|   IBIS Model for OMAP-L138ZWT
[IBIS Ver]   3.2
[Comment Char]  |_char
[File Name]   omapl138_zwt.ibs
[File Rev]   1.0
[Date]   March 8, 2013
[Source]   From Optimal Corporation's PakSi-E result.
[Notes]   Created from Freon_16x16_OSV_12172008_H_1.mcm
|   (1) OMAP-L138 ZWT contains dual rail I/O buffers that
|   are capable of running are two different core
|   voltages depedent on the schematic hookup
|   (a) 1.8V
|   (b) 3.3V
|   (2) Specific Model Sections/Name Decoders are determined
|   based upon the value that is supplied to the
|   particular I/O buffer as well as any pull up/down
|   resistors that are selected. Refer to the Model Selecter
|   Definitions for details regarding model selection at
|   1.8V rail or the 3.3V rail.
[Disclaimer]
|   Please be aware that in the absence of a written agreement
|   Texas Instruments (TI) assumes no liability for:
|   (1) The accuracy of the IBIS models provided to your company
|   (2) The proper functioning of these Models in your design
|   or for any resulting applications;or
|   (3) Infringement of patents,copyrights, or intellectual
|   property rights resulting from your use of these models.
|   TI provides IBIS Models as a service to our customers and
|   therefore reserves the right to limit distribution of the
|   Models.
[Copyright] Copyright 2011, Texas Instruments Incorporated. All Rights Reserved
[Component]   OMAP-L138ZWT
[Manufacturer]   Texas Instruments
[Package]
| variable   typ   min   max
R_pkg   4.82714e-001  2.28452e-002  7.70788e-001
L_pkg   4.49415e-009  1.01960e-010  8.14120e-009
C_pkg   9.77617e-013  6.27144e-013  1.43784e-012
[Pin] signal_name  model_name R_pin   L_pin   C_pin
| Note: Signal Name(s) may be truncated to meet the 80 character
|  per line limit. Refer to the IBIS Specification v3.2 for details
|   Name   I/O Model Name   R_pin  L_pin  C_pin
A1   ACLKR_PRU0_R3020  BC1833DV40CTPBFZ   6.70522e-001 7.77430e-009 1.18111e-012
B1   ACLKX_PRU0_R3019  BC1833DV40CTPBFZ   5.95613e-001 7.11870e-009 1.10755e-012
C2   AFSR_GP013   BC1833DV40CTPBFZ   5.89537e-001 6.09860e-009 1.05275e-012
B2   AFSX_GP012   BC1833DV40CTPBFZ   6.03424e-001 6.46010e-009 1.17554e-012
A2   AHCLKR_PRU0   BC1833DV40CTPBFZ   7.35160e-001 8.00800e-009 1.28347e-012
A3   AHCLKX_USB_REFCL  BC1833DV40CTPBFZ   6.42625e-001 7.06830e-009 1.36079e-012
D5   AMUTE_PRU0_R3016  BC1833DV40CTPBFZ   4.86289e-001 4.23260e-009 1.27108e-012
F4   RTCALARM_UART2CTS BC1833DV40CTPBFZ   2.81206e-001 2.78020e-009 1.04628e-012
F3   AXR0_ECAP0_APWM0  BC1833DV40CTPBFZ   4.75476e-001 4.39770e-009 9.49020e-013
E1   AXR1_DX0_GP19   BC1833DV40CTPBFZ   5.93339e-001 6.18190e-009 8.74765e-013
D4   AXR10_DR1_GP02   BC1833DV40CTPBFZ   4.51090e-001 3.95820e-009 1.11813e-012
C5   AXR11_FSX1_GP03   BC1833DV40CTPBFZ   3.47764e-001 4.08280e-009 1.06988e-012
C4   AXR12_FSR1_GP04   BC1833DV40CTPBFZ   5.63347e-001 5.37170e-009 1.17818e-012
B3   AXR13_CLKX1_GP05  BC1833DV40CTPBFZ   5.67122e-001 5.57030e-009 1.00192e-012
B4   AXR14_CLKR1_GP06  BC1833DV40CTPBFZ   5.99370e-001 6.02370e-009 1.15465e-012
A4   AXR15_EPWM0TZ0   BC1833DV40CTPBFZ   6.42602e-001 6.52960e-009 1.05664e-012
E2   AXR2_DR0_GP110   BC1833DV40CTPBFZ   5.58852e-001 5.75040e-009 9.93021e-013
E3   AXR3_FSX0_GP111   BC1833DV40CTPBFZ   5.43755e-001 5.35620e-009 1.08545e-012
D1   AXR4_FSR0_GP112   BC1833DV40CTPBFZ   6.02267e-001 6.21600e-009 9.81175e-013
D3   AXR5_CLKX0_GP113  BC1833DV40CTPBFZ   5.70240e-001 5.75810e-009 1.11536e-012
C1   AXR6_CLKR0_GP114  BC1833DV40CTPBFZ   6.53337e-001 6.85970e-009 1.03127e-012
D2   AXR7_EPWM1TZ0   BC1833DV40CTPBFZ   5.67627e-001 5.78120e-009 1.00529e-012
E4   AXR8_CLKS1_ECAP1  BC1833DV40CTPBFZ   6.23878e-001 5.57980e-009 1.16291e-012
C3   AXR9_DX1_GP01   BC1833DV40CTPBFZ   5.40131e-001 5.24750e-009 1.09974e-012
C14  EMAA0_GP50   BC1833DV40CTPBFZ   4.25288e-001 4.03200e-009 8.58918e-013
D15  EMAA1_GP51   BC1833DV40CTPBFZ   6.48857e-001 6.26150e-009 1.03443e-012
C12  EMAA10_PRU1R3018  BC1833DV40CTPBFZ   4.43266e-001 3.29860e-009 9.62048e-013
B12  EMAA11_PRU1R3019  BC1833DV40CTPBFZ   4.58807e-001 4.50390e-009 8.92001e-013
D13  EMAA12_PRU1R3020  BC1833DV40CTPBFZ   5.70361e-001 5.18860e-009 1.11139e-012
D11  EMAA13_PRU0R3021  BC1833DV40CTPBFZ   2.99405e-001 2.17920e-009 8.54180e-013
A12  EMAA14_MMCSD0DAT7 BC1833DV40CTPBFZ   4.83438e-001 4.55840e-009 8.59351e-013
C11  EMAA15_MMCSD0DAT6 BC1833DV40CTPBFZ   4.98593e-001 4.57870e-009 9.76252e-013
E12  EMAA16_MMCSD0DAT5 BC1833DV40CTPBFZ   5.62236e-001 4.38610e-009 1.25589e-012
B11  EMAA17_MMCSD0DAT4 BC1833DV40CTPBFZ   5.53553e-001 5.27900e-009 9.29416e-013
E11  EMAA18_MMCSD0DAT3 BC1833DV40CTPBFZ   4.25775e-001 3.44230e-009 1.11095e-012
C10  EMAA19_MMCSD0DAT2 BC1833DV40CTPBFZ   3.59339e-001 3.13160e-009 8.65773e-013
B14  EMAA2_GP52   BC1833DV40CTPBFZ   4.90044e-001 4.46920e-009 8.58488e-013
A11  EMAA20_MMCSD0DAT1 BC1833DV40CTPBFZ   5.00066e-001 4.69570e-009 8.08773e-013
B10  EMAA21_MMCSD0DAT0 BC1833DV40CTPBFZ   4.03175e-001 3.79000e-009 8.37205e-013
A10  EMAA22_MMCSD0CMD  BC1833DV40CTPBFZ   4.79165e-001 4.38050e-009 7.51561e-013
E9   MMCSD0CLK_GP47   BC1833DV40CTPBFZ   3.19355e-001 2.48480e-009 1.02209e-012
D14  EMAA3_GP53   BC1833DV40CTPBFZ   4.12224e-001 3.83380e-009 9.03674e-013
A14  EMAA4_GP54   BC1833DV40CTPBFZ   5.22455e-001 4.90270e-009 8.26256e-013
C13  EMAA5_GP55   BC1833DV40CTPBFZ   4.50260e-001 3.65480e-009 9.09443e-013
E13  EMAA6_GP56   BC1833DV40CTPBFZ   3.88312e-001 3.04460e-009 9.87596e-013
B13  EMAA7_PRU1R3015   BC1833DV40CTPBFZ   4.50502e-001 3.95110e-009 8.24200e-013
A13  EMAA8_PRU1R3016   BC1833DV40CTPBFZ   4.86150e-001 4.52080e-009 8.53585e-013
D12  EMAA9_PRU1R3017   BC1833DV40CTPBFZ   3.45739e-001 2.59770e-009 9.45330e-013
C15  EMABA0_GP28   BC1833DV40CTPBFZ   5.40104e-001 5.41780e-009 1.01378e-012
A15  EMABA1_GP29   BC1833DV40CTPBFZ   5.46634e-001 5.32220e-009 8.41073e-013
A9   EMACAS_PRU0R302   BC1833DV40CTPBFZ   4.68477e-001 4.48480e-009 7.79223e-013
B7   EMACLK_PRU0R305   BC1833DV40CTPBFZ   2.91044e-001 3.06540e-009 7.71567e-013
A18  EMACS0_GP20   BC1833DV40CTPBFZ   5.38591e-001 5.53120e-009 9.41554e-013
B17  EMACS2_GP315   BC1833DV40CTPBFZ   4.97514e-001 4.71050e-009 1.06659e-012
A17  EMACS3_GP314   BC1833DV40CTPBFZ   5.17167e-001 5.33980e-009 9.74323e-013
F9   EMA_CS4_GP313   BC1833DV40CTPBFZ   4.25846e-001 3.22730e-009 1.05377e-012
B16  EMA_CS5_GP312   BC1833DV40CTPBFZ   5.13656e-001 5.27280e-009 9.94069e-013
C9   EMA_D0_GP48   BC1833DV40CTPBFZ   2.94182e-001 2.42780e-009 7.80729e-013
A8   EMA_D1_GP49   BC1833DV40CTPBFZ   4.53721e-001 3.97270e-009 6.68142e-013
A7   EMA_D10_GP32   BC1833DV40CTPBFZ   4.53897e-001 4.01310e-009 6.27144e-013
D6   EMA_D11_GP33   BC1833DV40CTPBFZ   2.38604e-001 1.84040e-009 9.19954e-013
A6   EMA_D12_GP34   BC1833DV40CTPBFZ   6.07425e-001 6.23350e-009 1.06419e-012
B6   EMA_D13_GP35   BC1833DV40CTPBFZ   5.18704e-001 3.99570e-009 1.13613e-012
C7   EMA_D14_GP36   BC1833DV40CTPBFZ   5.42315e-001 4.44590e-009 1.15928e-012
E6   EMA_D15_GP37   BC1833DV40CTPBFZ   2.06956e-001 1.69280e-009 1.11364e-012
B8   EMA_D2_GP410   BC1833DV40CTPBFZ   4.73441e-001 3.98830e-009 7.85717e-013
E8   EMA_D3_GP411   BC1833DV40CTPBFZ   4.22749e-001 3.94410e-009 1.12372e-012
B5   EMA_D4_GP412   BC1833DV40CTPBFZ   4.51845e-001 3.85460e-009 8.63651e-013
E7   EMA_D5_GP413   BC1833DV40CTPBFZ   3.33586e-001 2.90310e-009 1.43784e-012
C6   EMA_D6_GP414   BC1833DV40CTPBFZ   4.96088e-001 3.85350e-009 1.08802e-012
D7   EMA_D7_GP415   BC1833DV40CTPBFZ   5.38361e-001 4.46010e-009 1.14437e-012
E10  EMA_D8_GP30   BC1833DV40CTPBFZ   4.32262e-001 3.32570e-009 1.05394e-012
D9   EMA_D9_GP31   BC1833DV40CTPBFZ   3.85347e-001 2.99080e-009 8.85071e-013
B15  EMA_OE_GP310   BC1833DV40CTPBFZ   4.72394e-001 4.44610e-009 9.78222e-013
A16  EMARAS_PRU0R303   BC1833DV40CTPBFZ   5.02224e-001 5.36240e-009 9.17657e-013
D10  EMA_A_RW_GP39   BC1833DV40CTPBFZ   4.33366e-001 3.89220e-009 1.09829e-012
D8   EMASDCKE_PRU0R304 BC1833DV40CTPBFZ   3.50532e-001 3.43390e-009 9.99262e-013
B18  EMAWAIT0_PRU0R300 BC1833DV40CTPBFZ   5.00826e-001 5.00220e-009 1.02162e-012
B19  EMAWAIT1_PRU0R301 BC1833DV40CTPBFZ   5.87512e-001 6.06000e-009 1.14362e-012
B9   EMAWE_GP311   BC1833DV40CTPBFZ   4.59931e-001 4.00200e-009 8.81437e-013
C8   EMAWEN_DQM0_GP23  BC1833DV40CTPBFZ   4.26501e-001 3.88670e-009 8.47385e-013
A5   EMAWEN_DQM1_GP22  BC1833DV40CTPBFZ   5.02300e-001 4.62500e-009 9.18201e-013
U7   DDR_A0   BSSTL18TCSCGPBFZ   4.45631e-001 3.19210e-009 8.01643e-013
T7   DDR_A1   BSSTL18TCSCGPBFZ   4.96539e-001 3.76940e-009 8.49415e-013
W6   DDR_A2   BSSTL18TCSCGPBFZ   4.96471e-001 4.42250e-009 7.26808e-013
V6   DDR_A3   BSSTL18TCSCGPBFZ   3.12088e-001 3.23310e-009 8.95189e-013
U5   DDR_A4   BSSTL18TCSCGPBFZ   5.26530e-001 4.12820e-009 9.39252e-013
V5   DDR_A5   BSSTL18TCSCGPBFZ   5.14992e-001 4.12960e-009 9.22902e-013
W5   DDR_A6   BSSTL18TCSCGPBFZ   5.19100e-001 4.88150e-009 7.93247e-013
U6   DDR_A7   BSSTL18TCSCGPBFZ   2.51410e-001 2.52800e-009 7.93128e-013
U4   DDR_A8   BSSTL18TCSCGPBFZ   6.12082e-001 5.53420e-009 1.02068e-012
T6   DDR_A9   BSSTL18TCSCGPBFZ   2.31771e-001 2.10850e-009 9.12907e-013
W4   DDR_A10   BSSTL18TCSCGPBFZ   5.78537e-001 5.31210e-009 8.57850e-013
T4   DDR_A11   BSSTL18TCSCGPBFZ   6.10590e-001 5.44020e-009 1.07076e-012
V4   DDR_A12   BSSTL18TCSCGPBFZ   5.44157e-001 4.83840e-009 8.98639e-013
T5   DDR_A13   BSSTL18TCSCGPBFZ   2.67446e-001 2.33590e-009 9.47633e-013
V8   DDR_BA0   BSSTL18TCSCGPBFZ   4.42216e-001 3.50310e-009 7.33337e-013
T9   DDR_BA1   BSSTL18TCSCGPBFZ   2.04349e-001 1.84940e-009 9.12926e-013
U8   DDR_BA2   BSSTL18TCSCGPBFZ   4.37893e-001 3.05980e-009 7.91011e-013
U9   DDR_CAS   BSSTL18TCSCGPBFZ   4.32382e-001 3.03600e-009 7.82466e-013
V7   DDR_CKE   BSSTL18TCSCGPBFZ   3.40193e-001 3.02880e-009 9.57595e-013
W7   DDR_CLKN   BSSTL18TCSCGPBFZ   4.87824e-001 4.14380e-009 7.11675e-013
W8   DDR_CLKP   BSSTL18TCSCGPBFZ   4.87706e-001 4.04160e-009 6.90005e-013
V9   DDR_CS   BSSTL18TCSCGPBFZ   4.22988e-001 3.32520e-009 7.05256e-013
U15  DDR_D0   BSSTL18TCSCGPBFZ   6.14599e-001 5.57430e-009 1.29241e-012
U14  DDR_D1   BSSTL18TCSCGPBFZ   6.77148e-001 6.88480e-009 1.15168e-012
V14  DDR_D2   BSSTL18TCSCGPBFZ   5.94668e-001 5.57310e-009 9.65300e-013
U13  DDR_D3   BSSTL18TCSCGPBFZ   6.42634e-001 6.44770e-009 1.01003e-012
V13  DDR_D4   BSSTL18TCSCGPBFZ   4.33037e-001 3.98350e-009 9.49332e-013
V12  DDR_D5   BSSTL18TCSCGPBFZ   5.17811e-001 4.36040e-009 8.60120e-013
W12  DDR_D6   BSSTL18TCSCGPBFZ   5.06957e-001 4.65170e-009 7.75559e-013
W11  DDR_D7   BSSTL18TCSCGPBFZ   3.40053e-001 3.84150e-009 8.42329e-013
T13  DDR_D8   BSSTL18TCSCGPBFZ   7.02824e-001 6.76610e-009 1.10155e-012
T11  DDR_D9   BSSTL18TCSCGPBFZ   5.38116e-001 4.19250e-009 9.33339e-013
T10  DDR_D10   BSSTL18TCSCGPBFZ   2.04836e-001 1.48950e-009 9.32683e-013
T12  DDR_D11   BSSTL18TCSCGPBFZ   5.39560e-001 4.18730e-009 9.72172e-013
U10  DDR_D12   BSSTL18TCSCGPBFZ   4.90524e-001 3.70090e-009 8.22331e-013
V10  DDR_D13   BSSTL18TCSCGPBFZ   5.08659e-001 4.15820e-009 8.09492e-013
U11  DDR_D14   BSSTL18TCSCGPBFZ   6.41945e-001 6.15820e-009 1.03041e-012
W10  DDR_D15   BSSTL18TCSCGPBFZ   3.34786e-001 3.81520e-009 1.10872e-012
W13  DDR_DQM0   BSSTL18TCSCGPBFZ   5.20588e-001 4.86740e-009 8.32828e-013
R10  DDR_DQM1   BSSTL18TCSCGPBFZ   5.83727e-001 4.04600e-009 1.10450e-012
W9   DDR_RAS   BSSTL18TCSCGPBFZ   4.85812e-001 4.18190e-009 7.68725e-013
R11  DDR_DQGATE0   BSSTL18TCSCGPBFZ   5.83676e-001 4.67250e-009 1.10827e-012
R12  DDR_DQGATE1   BSSTL18TCSCGPBFZ   6.09492e-001 4.92430e-009 1.16221e-012
T8   DDR_WE   BSSTL18TCSCGPBFZ   4.85661e-001 3.30550e-009 8.77513e-013
T14  DDR_DQS0   BSSTL18TCSCGPBFZ   5.56352e-001 4.85410e-009 1.06523e-012
V11  DDR_DQS1   BSSTL18TCSCGPBFZ   5.57030e-001 5.17590e-009 8.65934e-013
J16  EMU0   BC1833DV40CTPBFZ   2.69609e-001 2.51080e-009 9.18189e-013
K16  EMU1   BC1833DV40CTPBFZ   4.38711e-001 3.98660e-009 9.93256e-013
K4   PRU1R300_GP61   BC1833DV40CTPBFZ   3.74055e-001 3.00300e-009 9.72837e-013
J3   MMCSD1DAT1_GP62   BC1833DV40CTPBFZ   3.47731e-001 3.56010e-009 1.13728e-012
K3   MMCSD1DAT2_GP63   BC1833DV40CTPBFZ   4.24020e-001 3.61250e-009 8.08369e-013
H3   MMCSD1DAT3_GP64   BC1833DV40CTPBFZ   4.58330e-001 4.27570e-009 1.14982e-012
F2   MMCSD1DAT6_GP810  BC1833DV40CTPBFZ   6.57130e-001 6.53900e-009 1.00913e-012
F1   MMCSD1DAT7_GP811  BC1833DV40CTPBFZ   5.88435e-001 6.09970e-009 9.74970e-013
G3   PRU0R3022_GP812   BC1833DV40CTPBFZ   5.69940e-001 5.39570e-009 1.05523e-012
J4   PRU0R3023_GP813   BC1833DV40CTPBFZ   4.77184e-001 3.73550e-009 9.74249e-013
G2   PRU0R3024_GP814   BC1833DV40CTPBFZ   6.21314e-001 5.98450e-009 1.11595e-012
G1   PRU0R3025_GP815   BC1833DV40CTPBFZ   5.69099e-001 5.59150e-009 9.76024e-013
G4   MMCSD1DAT4_GP88   BC1833DV40CTPBFZ   4.94773e-001 4.21470e-009 9.49852e-013
H4   MMCSD1DAT5_GP89   BC1833DV40CTPBFZ   4.03091e-001 3.39770e-009 8.67477e-013
R5   GP60_PRU1_R3128   BC1833DV40CTPBFZ   2.17019e-001 2.01170e-009 1.03367e-012
W1   GP78_PRU1_R318   BC1833DV40CTPBFZ   6.10612e-001 6.27700e-009 1.06224e-012
W2   GP79_PRU1_R319   BC1833DV40CTPBFZ   6.30960e-001 6.09510e-009 1.07989e-012
T2   GP72_BOOT2   BC1833DV40CTPBFZ   5.01419e-001 4.54420e-009 9.41778e-013
T3   GP73_BOOT3   BC1833DV40CTPBFZ   4.48620e-001 3.96710e-009 1.00841e-012
R1   GP74_BOOT4   BC1833DV40CTPBFZ   5.49394e-001 5.30490e-009 8.92921e-013
R2   GP75_BOOT5   BC1833DV40CTPBFZ   5.25084e-001 4.72090e-009 9.30217e-013
R3   GP76_BOOT6   BC1833DV40CTPBFZ   3.55031e-001 4.19040e-009 1.05191e-012
P4   GP77_BOOT7   BC1833DV40CTPBFZ   4.27865e-001 3.34850e-009 9.06244e-013
W3   GP710_PRU1_R3110  BC1833DV40CTPBFZ   2.28452e-002 1.01960e-010 1.14444e-012
V1   GP711_PRU1_R3111  BC1833DV40CTPBFZ   6.46932e-001 6.50160e-009 9.88236e-013
V2   GP712_PRU1_R3112  BC1833DV40CTPBFZ   6.09370e-001 5.95910e-009 1.01546e-012
V3   GP713_PRU1_R3113  BC1833DV40CTPBFZ   5.28937e-001 5.19450e-009 1.02431e-012
U1   GP714_PRU1_R3114  BC1833DV40CTPBFZ   6.13427e-001 6.07030e-009 9.50946e-013
U2   GP715_PRU1_R3115  BC1833DV40CTPBFZ   5.67068e-001 5.44350e-009 9.82215e-013
U3   GP70_BOOT0   BC1833DV40CTPBFZ   5.43323e-001 4.88320e-009 9.28297e-013
T1   GP71_BOOT1   BC1833DV40CTPBFZ   5.55285e-001 5.17990e-009 8.95632e-013
J17  NMI   IC1833DVTPBFZP18LL 3.90575e-001 3.53870e-009 8.65772e-013
K14  RESET   IHHV1833DVTP18   2.72523e-001 1.96490e-009 1.01740e-012
K17  RTCK_GPIO80   BC1833DV40CTPBFZ   4.92642e-001 4.55900e-009 9.97242e-013
D19  SPI0CLK_EPWM0A   BC1833DV40CTPBFZ   4.59265e-001 4.70770e-009 8.79586e-013
C17  SPI0ENA_EPWM0B   BC1833DV40CTPBFZ   3.70510e-001 3.41200e-009 9.82922e-013
D17  SPI0SCS0_GP16   BC1833DV40CTPBFZ   4.89709e-001 4.51290e-009 9.79226e-013
E16  SPI0SCS1_GP17   BC1833DV40CTPBFZ   2.89181e-001 2.59760e-009 9.34814e-013
D16  SPI0SCS2_UART0RTS BC1833DV40CTPBFZ   3.74659e-001 3.47800e-009 1.02901e-012
E17  SPI0SCS3_UART0CTS BC1833DV40CTPBFZ   4.07379e-001 3.42510e-009 8.91820e-013
D18  SPI0SCS4_UART0TXD BC1833DV40CTPBFZ   4.05970e-001 4.12160e-009 9.47389e-013
C19  SPI0SCS5_UART0RXD BC1833DV40CTPBFZ   5.18855e-001 5.40240e-009 1.03877e-012
C18  SPI0SIMO_EPWMSYNO BC1833DV40CTPBFZ   4.65679e-001 4.70460e-009 9.61861e-013
C16  SPI0SOMI_EPWMSYNI BC1833DV40CTPBFZ   3.23590e-001 2.82350e-009 1.01704e-012
G19  SPI1CLK_GP213   BC1833DV40CTPBFZ   4.82388e-001 4.87790e-009 7.93438e-013
H16  SPI1ENA_GP212   BC1833DV40CTPBFZ   2.72059e-001 2.46120e-009 8.55327e-013
E19  SPI1SCS0_EPWM1B   BC1833DV40CTPBFZ   5.54124e-001 5.35800e-009 9.27298e-013
F18  SPI1SCS1_EPWM1A   BC1833DV40CTPBFZ   4.85756e-001 4.43690e-009 8.32222e-013
F19  SPI1SCS2_UART1TXD BC1833DV40CTPBFZ   5.30911e-001 5.08600e-009 7.97381e-013
E18  SPI1SCS3_UART1RXD BC1833DV40CTPBFZ   4.68304e-001 4.29180e-009 9.40515e-013
F16  SPI1SCS4_UART2TXD BC1833DV40CTPBFZ   3.84822e-001 3.09280e-009 8.50042e-013
F17  SPI1SCS5_UART2RXD BC1833DV40CTPBFZ   3.97204e-001 3.45760e-009 8.68842e-013
G18  SPI1SCS6_I2C0SDA  BC1833DV40CTPBFZ   4.36493e-001 3.97070e-009 8.05354e-013
G16  SPI1SCS7_I2C0SCL  BC1833DV40CTPBFZ   3.28582e-001 2.93800e-009 8.59756e-013
G17  SPI1SIMO_GP210   BC1833DV40CTPBFZ   4.15146e-001 3.62330e-009 7.78290e-013
H17  SPI1SOMI_GP211   BC1833DV40CTPBFZ   3.86238e-001 3.40470e-009 7.95949e-013
J15  TCK   IC1833DVTPBFZP18LL 2.72627e-001 2.07350e-009 9.10142e-013
M16  TDI   IC1833DVTPBFZP18LL 4.76009e-001 4.06980e-009 1.10114e-012
J18  TDO   BC1833DV40CTPBFZ   4.62219e-001 4.41060e-009 8.33533e-013
L16  TMS   IC1833DVTPBFZP18LL 4.14469e-001 3.71980e-009 9.85935e-013
L17  TRST   IC1833DVTPBFZP18LL 4.62541e-001 4.28940e-009 9.92132e-013
T17  RESETOUT_GP615   BC1833DV40CTPBFZ   3.51998e-001 3.17240e-009 1.08276e-012
U17  PRU0_R3029_GP611  BC1833DV40CTPBFZ   7.12182e-001 6.64690e-009 1.37972e-012
W15  PRU0_R3028_GP610  BC1833DV40CTPBFZ   5.66822e-001 5.43060e-009 8.83116e-013
W14  PRU1_R3010_GP67   BC1833DV40CTPBFZ   4.65680e-001 4.58120e-009 9.12942e-013
P17  GP65_PRU1_R310   BC1833DV40CTPBFZ   3.94808e-001 3.89780e-009 1.00392e-012
R15  PRU0R309_PRU0R319 BC1833DV40CTPBFZ   2.93369e-001 2.38090e-009 8.58888e-013
W17  RMIIRXER   BC1833DV40CTPBFZ   6.23033e-001 6.29800e-009 1.04906e-012
V17  RMIIRXD0   BC1833DV40CTPBFZ   6.63187e-001 6.71370e-009 1.15741e-012
W16  RMIIRXD1   BC1833DV40CTPBFZ   5.88099e-001 5.77390e-009 1.00930e-012
R14  RMIITXEN   BC1833DV40CTPBFZ   2.79926e-001 2.37250e-009 1.10763e-012
V16  RMIITXD0   BC1833DV40CTPBFZ   6.28546e-001 6.07180e-009 1.03347e-012
U18  RMIITXD1   BC1833DV40CTPBFZ   7.70788e-001 8.14120e-009 1.27165e-012
R19  PRU0R3010   BC1833DV40CTPBFZ   5.06077e-001 5.39890e-009 9.20909e-013
R18  PRU0R3011   BC1833DV40CTPBFZ   4.14016e-001 4.19930e-009 9.20996e-013
T16  PRU0R3012   BC1833DV40CTPBFZ   4.21661e-001 4.35600e-009 1.28119e-012
U19  PRU0R3013   BC1833DV40CTPBFZ   7.62887e-001 7.98930e-009 1.25280e-012
V19  PRU0R3014   BC1833DV40CTPBFZ   7.40621e-001 7.53910e-009 1.22918e-012
V18  PRU0R3015   BC1833DV40CTPBFZ   6.75889e-001 6.81150e-009 1.16111e-012
W19  RMIICRSDV   BC1833DV40CTPBFZ   7.15571e-001 7.47710e-009 1.14295e-012
W18  RMIIMHZ50CLK   BC1833DV40CTPBFZ   6.75324e-001 6.97490e-009 1.15470e-012
V15  PRU1R309_GP66   BC1833DV40CTPBFZ   3.14880e-001 3.37620e-009 8.48511e-013
T18  CLKOUT_PRU1R3013  BC1833DV40CTPBFZ   5.69140e-001 5.76560e-009 1.18406e-012
U16  PRU0R3027_GP69   BC1833DV40CTPBFZ   6.61452e-001 6.14510e-009 1.34409e-012
R16  PRU0R3030_GP612   BC1833DV40CTPBFZ   2.93246e-001 2.79150e-009 9.80397e-013
R17  PRU0R3031_GP613   BC1833DV40CTPBFZ   3.53134e-001 3.19990e-009 1.00158e-012
T15  PRU0R3026_GP68   BC1833DV40CTPBFZ   4.93409e-001 4.61210e-009 1.32672e-012
K18  USB0DRVVBUS   BC1833DV40CTPBFZ   4.38960e-001 4.19960e-009 8.67876e-013
E15  CVDD   POWER   10.7175e-003 0.10309e-009 11.8946e-012
G13  CVDD   POWER   10.7175e-003 0.10309e-009 11.8946e-012
G7   CVDD   POWER   10.7175e-003 0.10309e-009 11.8946e-012
G8   CVDD   POWER   10.7175e-003 0.10309e-009 11.8946e-012
H10  CVDD   POWER   10.7175e-003 0.10309e-009 11.8946e-012
H11  CVDD   POWER   10.7175e-003 0.10309e-009 11.8946e-012
H12  CVDD   POWER   10.7175e-003 0.10309e-009 11.8946e-012
H13  CVDD   POWER   10.7175e-003 0.10309e-009 11.8946e-012
H6   CVDD   POWER   10.7175e-003 0.10309e-009 11.8946e-012
H7   CVDD   POWER   10.7175e-003 0.10309e-009 11.8946e-012
J12  CVDD   POWER   10.7175e-003 0.10309e-009 11.8946e-012
J6   CVDD   POWER   10.7175e-003 0.10309e-009 11.8946e-012
K12  CVDD   POWER   10.7175e-003 0.10309e-009 11.8946e-012
K6   CVDD   POWER   10.7175e-003 0.10309e-009 11.8946e-012
L12  CVDD   POWER   10.7175e-003 0.10309e-009 11.8946e-012
M8   CVDD   POWER   10.7175e-003 0.10309e-009 11.8946e-012
M9   CVDD   POWER   10.7175e-003 0.10309e-009 11.8946e-012
N8   CVDD   POWER   10.7175e-003 0.10309e-009 11.8946e-012
N10  DDR_DVDD18   POWER   44.8272e-003 0.27004e-009 4.07721e-012
N6   DDR_DVDD18   POWER   44.8272e-003 0.27004e-009 4.07721e-012
N9   DDR_DVDD18   POWER   44.8272e-003 0.27004e-009 4.07721e-012
P10  DDR_DVDD18   POWER   44.8272e-003 0.27004e-009 4.07721e-012
P7   DDR_DVDD18   POWER   44.8272e-003 0.27004e-009 4.07721e-012
P8   DDR_DVDD18   POWER   44.8272e-003 0.27004e-009 4.07721e-012
P9   DDR_DVDD18   POWER   44.8272e-003 0.27004e-009 4.07721e-012
R7   DDR_DVDD18   POWER   44.8272e-003 0.27004e-009 4.07721e-012
R8   DDR_DVDD18   POWER   44.8272e-003 0.27004e-009 4.07721e-012
R9   DDR_DVDD18   POWER   44.8272e-003 0.27004e-009 4.07721e-012
R6   DDR_VREF   NC
U12  DDR_ZP   NC
F14  DVDD18   POWER   21.9546e-003 0.15546e-009 7.95208e-012
G10  DVDD18   POWER   21.9546e-003 0.15546e-009 7.95208e-012
G11  DVDD18   POWER   21.9546e-003 0.15546e-009 7.95208e-012
G12  DVDD18   POWER   21.9546e-003 0.15546e-009 7.95208e-012
G6   DVDD18   POWER   21.9546e-003 0.15546e-009 7.95208e-012
J13  DVDD18   POWER   21.9546e-003 0.15546e-009 7.95208e-012
K5   DVDD18   POWER   21.9546e-003 0.15546e-009 7.95208e-012
L6   DVDD18   POWER   21.9546e-003 0.15546e-009 7.95208e-012
P13  DVDD18   POWER   21.9546e-003 0.15546e-009 7.95208e-012
R13  DVDD18   POWER   21.9546e-003 0.15546e-009 7.95208e-012
F15  DVDD3318_A   POWER
F5   DVDD3318_A   POWER
G14  DVDD3318_A   POWER
G15  DVDD3318_A   POWER
G5   DVDD3318_A   POWER
H5   DVDD3318_A   POWER
E14  DVDD3318_B   POWER
F10  DVDD3318_B   POWER
F11  DVDD3318_B   POWER
F12  DVDD3318_B   POWER
F13  DVDD3318_B   POWER
F6   DVDD3318_B   POWER
F7   DVDD3318_B   POWER
F8   DVDD3318_B   POWER
G9   DVDD3318_B   POWER
J14  DVDD3318_B   POWER
K15  DVDD3318_B   POWER
J5   DVDD3318_C   POWER
K13  DVDD3318_C   POWER
L13  DVDD3318_C   POWER
L4   DVDD3318_C   POWER
M13  DVDD3318_C   POWER
N13  DVDD3318_C   POWER
P12  DVDD3318_C   POWER
P5   DVDD3318_C   POWER
P6   DVDD3318_C   POWER
R4   DVDD3318_C   POWER
M14  NC   NC
M3   NC   NC
N16  NC   NC
L19  OSCIN   NC
K19  OSCOUT   NC
L18  OSCVSS   GND
L15  PLL0_VDDA   POWER   243.028e-003 1.68968e-009 0.706515e-012
M17  PLL0_VSSA   GND
N15  PLL1_VDDA   POWER   357.761e-003 2.39647e-009 0.906375e-012
M15  PLL1_VSSA   GND
T19  RSV2   POWER
L14  RTC_CVDD   POWER   187.448e-003 1.48213e-009 0.648117e-012
H18  RTC_VSS   GND
J19  RTC_XI   NC
H19  RTC_XO   NC
E5   RVDD   POWER
H14  RVDD   POWER
N7   RVDD   POWER
N1   NC   NC
N2   NC   NC
N3   NC   NC
L2   NC   NC
L1   NC   NC
J2   NC   NC
J1   NC   NC
M2   NC   NC
N4   NC   NC
P1   NC   NC
P2   NC   NC
P3   NC   NC
H1   VSS   GND
H2   VSS   GND
K1   VSS   GND
K2   VSS   GND
L3   VSS   GND
M1   VSS   GND
M12  USB_CVDD   POWER   373.588e-003 3.31393e-009 0.61952e-012
M18  USB0_DM   NC
M19  USB0_DP   NC
P16  USB0_ID   NC
N19  USB0_VBUS   NC
N17  USB0_VDDA12   POWER
N14  USB0_VDDA18   POWER   264.320e-003 1.9838e-009 0.742393e-012
N18  USB0_VDDA33   POWER   599.405e-003 4.8937e-009 0.786878e-012
P18  NC   NC
P19  NC   NC
P14  NC   POWER
P15  NC   POWER
A19  VSS   GND
H15  VSS   GND
H8   VSS   GND
H9   VSS   GND
J10  VSS   GND
J11  VSS   GND
J7   VSS   GND
J8   VSS   GND
J9   VSS   GND
K10  VSS   GND
K11  VSS   GND
K7   VSS   GND
K8   VSS   GND
K9   VSS   GND
L10  VSS   GND
L11  VSS   GND
L5   VSS   GND
L7   VSS   GND
L8   VSS   GND
L9   VSS   GND
M10  VSS   GND
M11  VSS   GND
M4   VSS   GND
M5   VSS   GND
M6   VSS   GND
M7   VSS   GND
N11  VSS   GND
N12  VSS   GND
N5   VSS   GND
P11  VSS   GND
[Model Selector] IHHV1833DVTP18
|  This seciton is used to determine the IBIS model to use depending
|  on which voltage is supplied to the Dual Voltage I/O Buffers
HV1833DVTP18_7LM_1P8   Dual Voltage I/O Buffer with 1.8V External Supply
HV1833DVTP18_7LM_3P3   Dual Voltage I/O Buffer with 3.3V External Supply
[Model Selector] IC1833DVTPBFZP18LL
|  This seciton is used to determine which IBIS Model is to be used
|  for the pins depending on the functionality required by the user's
|  application.
BFZP18LL_!PI_LOW_1P8  Cell operated at 1.8(nom)
|IC1833DVTPBFZP18LL_!PI_LOW_1P8;
|BUFFER WITH WEAK_PULLDOWN_ON NOMINAL CURRENT OF 100UA WHEN PAD=VDDS
FZP18LL_!PI_HIGH_1P8  Cell operated at 1.8(nom)
|IC1833DVTPBFZP18LL_!PI_HIGH_1P8;
|BUFFER WITH WEAK_PULLUP_ON NOMINAL CURRENT OF 100UA WHEN PAD=0
3DVTPBFZP18LL_PI_1P8  Cell operated at 1.8(nom)
|IC1833DVTPBFZP18LL_PI_1P8;
|BUFFER IN NORMAL MODE WITH PULLUP AND PULLDOWN OFF
BFZP18LL_!PI_LOW_3P3  Cell operated at 3.3(nom)
|IC1833DVTPBFZP18LL_!PI_LOW_3P3;
|BUFFER WITH WEAK_PULLDOWN_ON NOMINAL CURRENT OF 100UA WHEN PAD=VDDS
FZP18LL_!PI_HIGH_3P3  Cell operated at 3.3(nom)
|IC1833DVTPBFZP18LL_!PI_HIGH_3P3;
|BUFFER WITH WEAK_PULLUP_ON NOMINAL CURRENT OF 100UA WHEN PAD=0
3DVTPBFZP18LL_PI_3P3  Cell operated at 3.3(nom)
|IC1833DVTPBFZP18LL_PI_3P3;
|BUFFER IN NORMAL MODE WITH PULLUP AND PULLDOWN OFF
[Model Selector] BC1833DV40CTPBFZ
|  This seciton is used to determine the IBIS model to use depending
|  on which voltage is supplied to the Dual Voltage I/O Buffers
18LL_X50_!PI_LOW_1P8  Cell operated at 1.8(nom)
|BC1833DV40CTPBFZ_!PI_LOW_1P8;
|BUFFER WITH WEAK_PULLDOWN_ON NOMINAL CURRENT OF 100UA WHEN PAD=VDDS
8LL_X50_!PI_HIGH_1P8  Cell operated at 1.8(nom)
|BC1833DV40CTPBFZ_!PI_HIGH_1P8;
|BUFFER WITH WEAK_PULLUP_ON NOMINAL CURRENT OF 100UA WHEN PAD=0
PBFZP18LL_X50_PI_1P8  Cell operated at 1.8(nom)
|BC1833DV40CTPBFZ_PI_1P8;
|BUFFER IN NORMAL MODE WITH PULLUP AND PULLDOWN OFF
18LL_X50_!PI_LOW_3P3  Cell operated at 3.3(nom)
|BC1833DV40CTPBFZ_!PI_LOW_3P3;
|BUFFER WITH WEAK_PULLDOWN_ON NOMINAL CURRENT OF 100UA WHEN PAD=VDDS
8LL_X50_!PI_HIGH_3P3  Cell operated at 3.3(nom)
|BC1833DV40CTPBFZ_!PI_HIGH_3P3;
|BUFFER WITH WEAK_PULLUP_ON NOMINAL CURRENT OF 100UA WHEN PAD=0
PBFZP18LL_X50_PI_3P3  Cell operated at 3.3(nom)
|BC1833DV40CTPBFZ_PI_3P3;
|BUFFER IN NORMAL MODE WITH PULLUP AND PULLDOWN OFF
[Model Selector] BSSTL18TCSCGPBFZ
NOSR0_NOTERM_1P8  Cell operated at 1.8(nom)
|NOSR0_NOTERM_1P8
|BUFFER OPERATING AT FAST MODE WITH 1.8V SUPPLY WITH +/-10% VARIATION
NOSR0_NOTERM_0.1_1P8  Cell operated at 1.8(nom)
| Models and submodels in the file (16): HV1833DVTP18_7LM_1P8 (Input), HV1833DVTP18_7LM_3P3 (Input), BFZP18LL_!PI_LOW_1P8 (Input), FZP18LL_!PI_HIGH_1P8 (Input), 3DVTPBFZP18LL_PI_1P8 (Input), BFZP18LL_!PI_LOW_3P3 (Input), FZP18LL_!PI_HIGH_3P3 (Input), 3DVTPBFZP18LL_PI_3P3 (Input), NOSR0_NOTERM_1P8 (3-state), NOSR0_NOTERM_0.1_1P8 (3-state), 18LL_X50_!PI_LOW_1P8 (I/O), 8LL_X50_!PI_HIGH_1P8 (I/O), PBFZP18LL_X50_PI_1P8 (I/O), 18LL_X50_!PI_LOW_3P3 (I/O), 8LL_X50_!PI_HIGH_3P3 (I/O), PBFZP18LL_X50_PI_3P3 (I/O)
